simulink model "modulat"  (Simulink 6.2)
settings: Solver=ode45  StartTime=0.0  StopTime=5  MaxStep=0.001  MinStep=0.0001  RelTol=1e-3

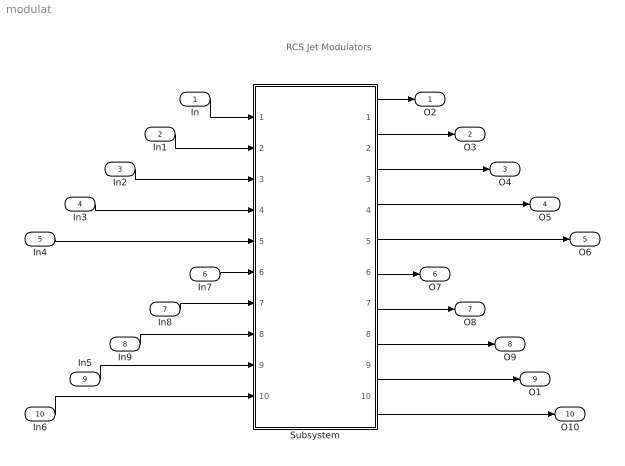
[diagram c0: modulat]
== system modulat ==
  note: RCS Jet Modulators
  In : Inport  Port=1  LatchInput=off
  In1 : Inport  Port=2  LatchInput=off
  In2 : Inport  Port=3  LatchInput=off
  In3 : Inport  Port=4  LatchInput=off
  In4 : Inport  Port=5  LatchInput=off
  In7 : Inport  Port=6  LatchInput=off
  In8 : Inport  Port=7  LatchInput=off
  In9 : Inport  Port=8  LatchInput=off
  In5 : Inport  Port=9  LatchInput=off
  In6 : Inport  Port=10  LatchInput=off
  Subsystem : Subsystem
  O2 : Outport
  O3 : Outport  Port=2
  O4 : Outport  Port=3
  O5 : Outport  Port=4
  O6 : Outport  Port=5
  O7 : Outport  Port=6
  O8 : Outport  Port=7
  O9 : Outport  Port=8
  O1 : Outport  Port=9
  O10 : Outport  Port=10
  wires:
  In/1 -> Subsystem/1(In)
  In1/1 -> Subsystem/2(In1)
  In2/1 -> Subsystem/3(In2)
  In3/1 -> Subsystem/4(In3)
  In4/1 -> Subsystem/5(In4)
  In7/1 -> Subsystem/6(In5)
  In8/1 -> Subsystem/7(In6)
  In9/1 -> Subsystem/8(In7)
  In5/1 -> Subsystem/9(In8)
  In6/1 -> Subsystem/10(In9)
  Subsystem/1(O) -> O2/1
  Subsystem/2(O1) -> O3/1
  Subsystem/3(O2) -> O4/1
  Subsystem/4(O3) -> O5/1
  Subsystem/5(O4) -> O6/1
  Subsystem/6(O5) -> O7/1
  Subsystem/7(O6) -> O8/1
  Subsystem/8(O7) -> O9/1
  Subsystem/10(O9) -> O10/1
  Subsystem/9(O8) -> O1/1

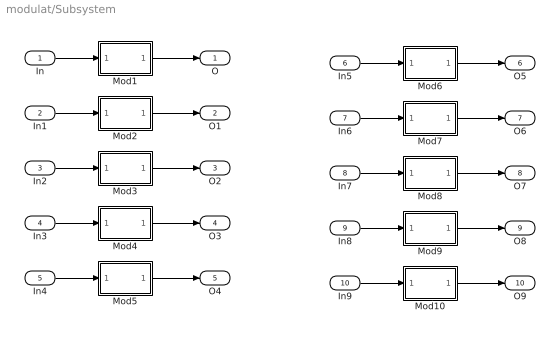
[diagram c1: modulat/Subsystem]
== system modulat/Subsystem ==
  In : Inport  Port=1  LatchInput=off
  In1 : Inport  Port=2  LatchInput=off
  In2 : Inport  Port=3  LatchInput=off
  In3 : Inport  Port=4  LatchInput=off
  In4 : Inport  Port=5  LatchInput=off
  In5 : Inport  Port=6  LatchInput=off
  In6 : Inport  Port=7  LatchInput=off
  In7 : Inport  Port=8  LatchInput=off
  In8 : Inport  Port=9  LatchInput=off
  In9 : Inport  Port=10  LatchInput=off
  Mod1 : Subsystem
  Mod10 : Subsystem
  Mod2 : Subsystem
  Mod3 : Subsystem
  Mod4 : Subsystem
  Mod5 : Subsystem
  Mod6 : Subsystem
  Mod7 : Subsystem
  Mod8 : Subsystem
  Mod9 : Subsystem
  O : Outport
  O1 : Outport  Port=2
  O2 : Outport  Port=3
  O3 : Outport  Port=4
  O4 : Outport  Port=5
  O5 : Outport  Port=6
  O6 : Outport  Port=7
  O7 : Outport  Port=8
  O8 : Outport  Port=9
  O9 : Outport  Port=10
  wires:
  In/1 -> Mod1/1(In1)
  Mod1/1(O1) -> O/1
  In1/1 -> Mod2/1(In1)
  Mod2/1(O1) -> O1/1
  In2/1 -> Mod3/1(In1)
  Mod3/1(O1) -> O2/1
  In3/1 -> Mod4/1(In1)
  Mod4/1(O1) -> O3/1
  In4/1 -> Mod5/1(In1)
  Mod5/1(O1) -> O4/1
  In5/1 -> Mod6/1(In1)
  Mod6/1(O1) -> O5/1
  In6/1 -> Mod7/1(In1)
  Mod7/1(O1) -> O6/1
  In7/1 -> Mod8/1(In1)
  Mod8/1(O1) -> O7/1
  In8/1 -> Mod9/1(In1)
  Mod9/1(O1) -> O8/1
  In9/1 -> Mod10/1(In1)
  Mod10/1(O1) -> O9/1

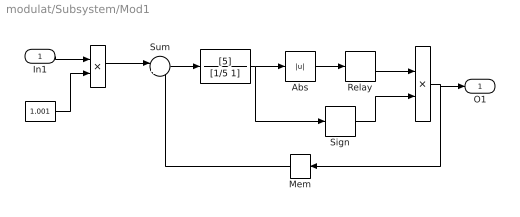
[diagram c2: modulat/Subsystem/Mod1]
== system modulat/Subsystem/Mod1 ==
  In1 : Inport  Port=1  LatchInput=off
  " " : Product
  "  " : TransferFcn  Numerator=[5]  Denominator=[1/5 1]
  "   " : Constant  Value=1.001
  "    " : Product
  Abs : Abs
  Mem : Memory  Orientation=left
  Relay : Relay  OnSwitchValue=0.5  OffSwitchValue=0.5
  Sign : Signum
  Sum : Sum  Inputs=|+-
  O1 : Outport
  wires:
  " "/1 -> Sum/1
  "   "/1 -> " "/2
  Sum/1 -> "  "/1
  "  "/1 -> Abs/1, Sign/1
  Abs/1 -> Relay/1
  Relay/1 -> "    "/1
  Sign/1 -> "    "/2
  Mem/1 -> Sum/2
  "    "/1 -> Mem/1, O1/1
  In1/1 -> " "/1

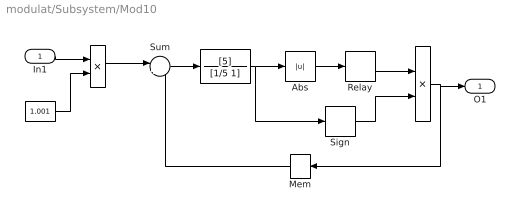
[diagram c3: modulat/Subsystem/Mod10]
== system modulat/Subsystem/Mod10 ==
  In1 : Inport  Port=1  LatchInput=off
  " " : Product
  "  " : TransferFcn  Numerator=[5]  Denominator=[1/5 1]
  "   " : Constant  Value=1.001
  "    " : Product
  Abs : Abs
  Mem : Memory  Orientation=left
  Relay : Relay  OnSwitchValue=0.5  OffSwitchValue=0.5
  Sign : Signum
  Sum : Sum  Inputs=|+-
  O1 : Outport
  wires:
  " "/1 -> Sum/1
  "   "/1 -> " "/2
  Sum/1 -> "  "/1
  "  "/1 -> Abs/1, Sign/1
  Abs/1 -> Relay/1
  Relay/1 -> "    "/1
  Sign/1 -> "    "/2
  Mem/1 -> Sum/2
  "    "/1 -> Mem/1, O1/1
  In1/1 -> " "/1

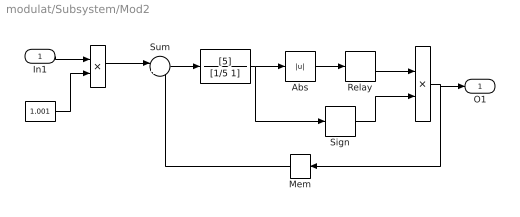
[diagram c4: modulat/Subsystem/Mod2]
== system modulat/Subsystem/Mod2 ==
  In1 : Inport  Port=1  LatchInput=off
  " " : Product
  "  " : TransferFcn  Numerator=[5]  Denominator=[1/5 1]
  "   " : Constant  Value=1.001
  "    " : Product
  Abs : Abs
  Mem : Memory  Orientation=left
  Relay : Relay  OnSwitchValue=0.5  OffSwitchValue=0.5
  Sign : Signum
  Sum : Sum  Inputs=|+-
  O1 : Outport
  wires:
  " "/1 -> Sum/1
  "   "/1 -> " "/2
  Sum/1 -> "  "/1
  "  "/1 -> Abs/1, Sign/1
  Abs/1 -> Relay/1
  Relay/1 -> "    "/1
  Sign/1 -> "    "/2
  Mem/1 -> Sum/2
  "    "/1 -> Mem/1, O1/1
  In1/1 -> " "/1

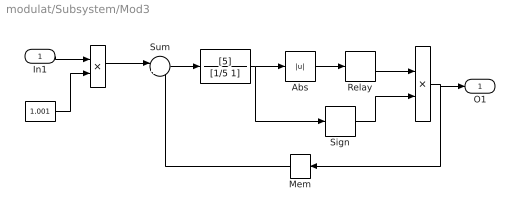
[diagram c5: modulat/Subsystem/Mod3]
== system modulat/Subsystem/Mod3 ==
  In1 : Inport  Port=1  LatchInput=off
  " " : Product
  "  " : TransferFcn  Numerator=[5]  Denominator=[1/5 1]
  "   " : Constant  Value=1.001
  "    " : Product
  Abs : Abs
  Mem : Memory  Orientation=left
  Relay : Relay  OnSwitchValue=0.5  OffSwitchValue=0.5
  Sign : Signum
  Sum : Sum  Inputs=|+-
  O1 : Outport
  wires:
  " "/1 -> Sum/1
  "   "/1 -> " "/2
  Sum/1 -> "  "/1
  "  "/1 -> Abs/1, Sign/1
  Abs/1 -> Relay/1
  Relay/1 -> "    "/1
  Sign/1 -> "    "/2
  Mem/1 -> Sum/2
  "    "/1 -> Mem/1, O1/1
  In1/1 -> " "/1

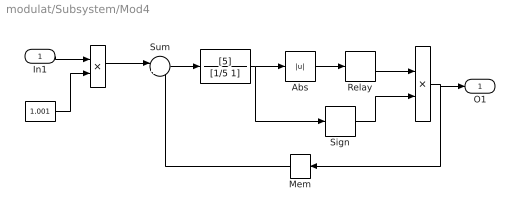
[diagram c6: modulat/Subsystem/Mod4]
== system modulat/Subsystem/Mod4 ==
  In1 : Inport  Port=1  LatchInput=off
  " " : Product
  "  " : TransferFcn  Numerator=[5]  Denominator=[1/5 1]
  "   " : Constant  Value=1.001
  "    " : Product
  Abs : Abs
  Mem : Memory  Orientation=left
  Relay : Relay  OnSwitchValue=0.5  OffSwitchValue=0.5
  Sign : Signum
  Sum : Sum  Inputs=|+-
  O1 : Outport
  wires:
  " "/1 -> Sum/1
  "   "/1 -> " "/2
  Sum/1 -> "  "/1
  "  "/1 -> Abs/1, Sign/1
  Abs/1 -> Relay/1
  Relay/1 -> "    "/1
  Sign/1 -> "    "/2
  Mem/1 -> Sum/2
  "    "/1 -> Mem/1, O1/1
  In1/1 -> " "/1

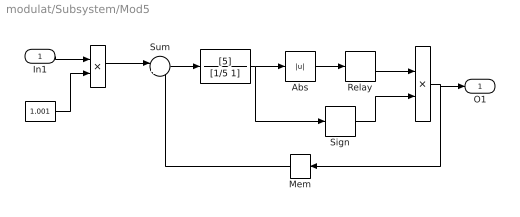
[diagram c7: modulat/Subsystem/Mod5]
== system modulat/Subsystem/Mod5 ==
  In1 : Inport  Port=1  LatchInput=off
  " " : Product
  "  " : TransferFcn  Numerator=[5]  Denominator=[1/5 1]
  "   " : Constant  Value=1.001
  "    " : Product
  Abs : Abs
  Mem : Memory  Orientation=left
  Relay : Relay  OnSwitchValue=0.5  OffSwitchValue=0.5
  Sign : Signum
  Sum : Sum  Inputs=|+-
  O1 : Outport
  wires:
  " "/1 -> Sum/1
  "   "/1 -> " "/2
  Sum/1 -> "  "/1
  "  "/1 -> Abs/1, Sign/1
  Abs/1 -> Relay/1
  Relay/1 -> "    "/1
  Sign/1 -> "    "/2
  Mem/1 -> Sum/2
  "    "/1 -> Mem/1, O1/1
  In1/1 -> " "/1

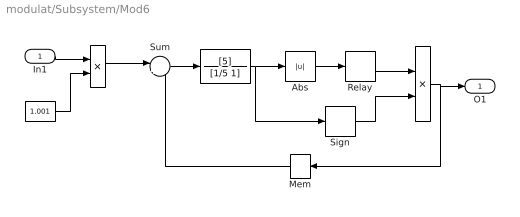
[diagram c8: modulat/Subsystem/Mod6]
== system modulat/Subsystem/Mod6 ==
  In1 : Inport  Port=1  LatchInput=off
  " " : Product
  "  " : TransferFcn  Numerator=[5]  Denominator=[1/5 1]
  "   " : Constant  Value=1.001
  "    " : Product
  Abs : Abs
  Mem : Memory  Orientation=left
  Relay : Relay  OnSwitchValue=0.5  OffSwitchValue=0.5
  Sign : Signum
  Sum : Sum  Inputs=|+-
  O1 : Outport
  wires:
  " "/1 -> Sum/1
  "   "/1 -> " "/2
  Sum/1 -> "  "/1
  "  "/1 -> Abs/1, Sign/1
  Abs/1 -> Relay/1
  Relay/1 -> "    "/1
  Sign/1 -> "    "/2
  Mem/1 -> Sum/2
  "    "/1 -> Mem/1, O1/1
  In1/1 -> " "/1

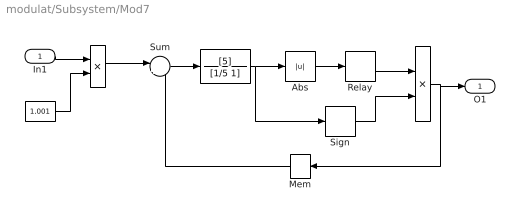
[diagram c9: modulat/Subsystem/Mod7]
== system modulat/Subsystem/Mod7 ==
  In1 : Inport  Port=1  LatchInput=off
  " " : Product
  "  " : TransferFcn  Numerator=[5]  Denominator=[1/5 1]
  "   " : Constant  Value=1.001
  "    " : Product
  Abs : Abs
  Mem : Memory  Orientation=left
  Relay : Relay  OnSwitchValue=0.5  OffSwitchValue=0.5
  Sign : Signum
  Sum : Sum  Inputs=|+-
  O1 : Outport
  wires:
  " "/1 -> Sum/1
  "   "/1 -> " "/2
  Sum/1 -> "  "/1
  "  "/1 -> Abs/1, Sign/1
  Abs/1 -> Relay/1
  Relay/1 -> "    "/1
  Sign/1 -> "    "/2
  Mem/1 -> Sum/2
  "    "/1 -> Mem/1, O1/1
  In1/1 -> " "/1

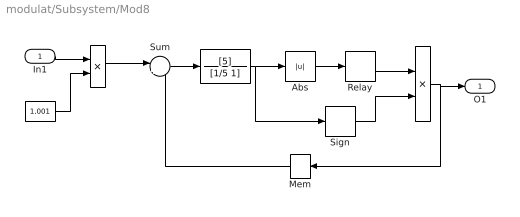
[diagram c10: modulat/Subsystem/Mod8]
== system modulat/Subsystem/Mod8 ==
  In1 : Inport  Port=1  LatchInput=off
  " " : Product
  "  " : TransferFcn  Numerator=[5]  Denominator=[1/5 1]
  "   " : Constant  Value=1.001
  "    " : Product
  Abs : Abs
  Mem : Memory  Orientation=left
  Relay : Relay  OnSwitchValue=0.5  OffSwitchValue=0.5
  Sign : Signum
  Sum : Sum  Inputs=|+-
  O1 : Outport
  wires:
  " "/1 -> Sum/1
  "   "/1 -> " "/2
  Sum/1 -> "  "/1
  "  "/1 -> Abs/1, Sign/1
  Abs/1 -> Relay/1
  Relay/1 -> "    "/1
  Sign/1 -> "    "/2
  Mem/1 -> Sum/2
  "    "/1 -> Mem/1, O1/1
  In1/1 -> " "/1

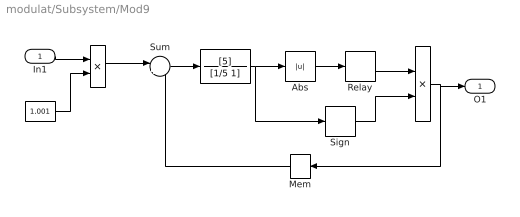
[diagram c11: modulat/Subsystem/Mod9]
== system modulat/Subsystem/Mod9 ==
  In1 : Inport  Port=1  LatchInput=off
  " " : Product
  "  " : TransferFcn  Numerator=[5]  Denominator=[1/5 1]
  "   " : Constant  Value=1.001
  "    " : Product
  Abs : Abs
  Mem : Memory  Orientation=left
  Relay : Relay  OnSwitchValue=0.5  OffSwitchValue=0.5
  Sign : Signum
  Sum : Sum  Inputs=|+-
  O1 : Outport
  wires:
  " "/1 -> Sum/1
  "   "/1 -> " "/2
  Sum/1 -> "  "/1
  "  "/1 -> Abs/1, Sign/1
  Abs/1 -> Relay/1
  Relay/1 -> "    "/1
  Sign/1 -> "    "/2
  Mem/1 -> Sum/2
  "    "/1 -> Mem/1, O1/1
  In1/1 -> " "/1
